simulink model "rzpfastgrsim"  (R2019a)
settings: configuration reference "configurationSettings" (kept in a data dictionary, not in this file)
undefined symbols (not defined in the file or in its folder): dtsimdata, TP

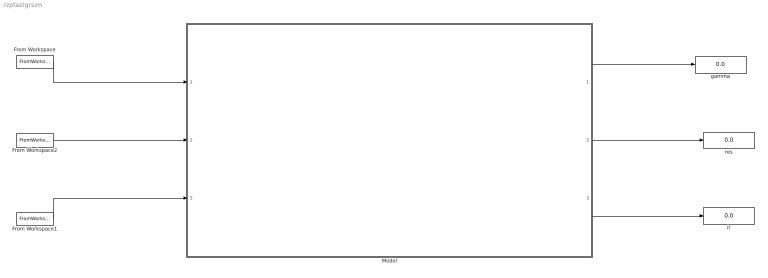
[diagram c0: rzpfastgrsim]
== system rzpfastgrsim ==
  From Workspace : FromWorkspace  VariableName=Ie  SampleTime=dtsimdata  Interpolate=off  OutputAfterFinalValue=Holding final value
  From Workspace1 : FromWorkspace  VariableName=Ip  SampleTime=dtsimdata  Interpolate=off  OutputAfterFinalValue=Holding final value
  From Workspace2 : FromWorkspace  VariableName=Iy  SampleTime=dtsimdata  Interpolate=off  OutputAfterFinalValue=Holding final value
  Model : ModelReference  ModelNameDialog=rzpfastgrslx.slx  SimulationMode=Normal  ModelReferenceVersion=1.90  mask{TP=TP}
  gamma : Display
  it : Display
  res : Display
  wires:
  Model/3 -> it/1
  Model/2 -> res/1
  Model/1 -> gamma/1
  From Workspace/1 -> Model/1
  From Workspace1/1 -> Model/3
  From Workspace2/1 -> Model/2
